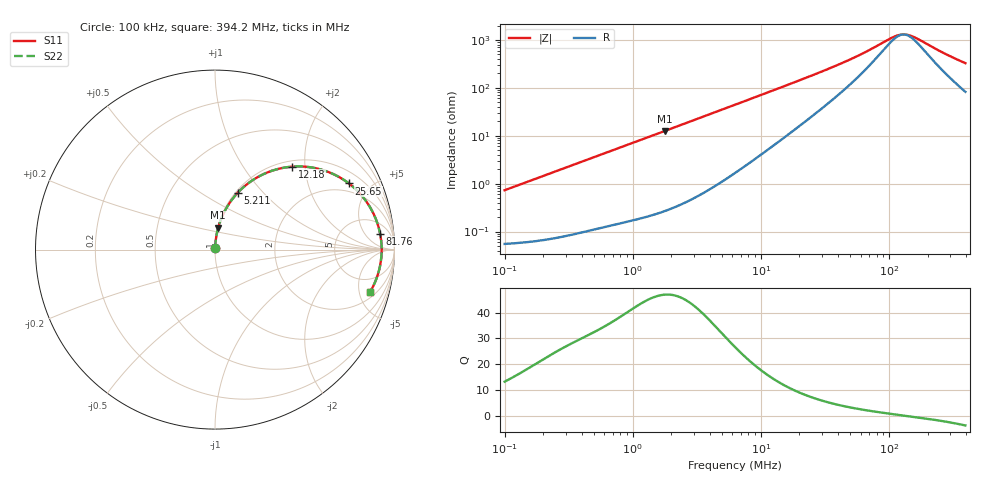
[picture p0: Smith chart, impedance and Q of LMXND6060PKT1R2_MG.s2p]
! LMXND6060PKT1R2_MG  S-PARAMETER MODEL  ( General Type )
! Model Generated by TAIYO YUDEN Corporation (https://www.yuden.co.jp/en/)
! Version 1.0
! TAIYO YUDEN Control No. 191025NI43SB-FBB
! Copyright(c) 2019 TAIYO YUDEN CO.,LTD. All Rights Reserved.
! Product Description (link to TY-COMPAS)
! https://ds.yuden.co.jp/TYCOMPAS/or/detail?pn=LMXND6060PKT1R2NMG&u=M
! Products Name : Inductors
! Characteristics :
!  Inductance : 1.2 uH , SRF(min) : 77 MHz , DC Resistance(max) : 0.0504 Ohm
!  Rated Current : Saturation :4000 mA , Temp Rise : 2750 mA (40 degC)
!  Case Size : 6.0 x 6.0 / 0.236 x 0.236 [mm/inch] , Thickness : 1.4 / 0.055 [mm/inch]
!  (Conditions: Temperature = 25 degC , DC Bias Current/Voltage = 0A / 0V)
! External Node Assignments :
!  1  o---GGG---o  2
! GND o---------o GND
! Frequency Range : 0.1MHz  -  394.189695MHz  [ 402 STEP ]
# MHz S RI R 50
! Freq[MHz].  S11 Real  S11 Imag  S21 Real  S21 Imag  S12 Real  S12 Imag  S22 Real  S22 Imag
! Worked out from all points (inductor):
!   401 points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, 100 kHz to 394.2 MHz, reference 50 ohm
!   read as one part in series: L = 1.15 uH near 104.2 kHz
!   highest Q = 47 at 1.776 MHz (marker M1), where L = 1.12 uH
!   self-resonance near 129.9 MHz
!   S11 on the Smith chart (normalised r, x): 100 kHz: 1.00, +0.01; 5.211 MHz: 1.02, +0.73; 12.18 MHz: 1.12, +1.72; 25.65 MHz: 1.54, +3.68; 81.76 MHz: 10, +12; 394.2 MHz: 2.65, -6.33
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0.1  0.000603 0.00724  0.9994 -0.00724  0.9994 -0.00724  0.000603 0.00724
0.400203  0.00177 0.0286  0.9982 -0.0286  0.9982 -0.0286  0.00177 0.0286
0.860763  0.00524 0.0606  0.9948 -0.0606  0.9948 -0.0606  0.00524 0.0606
1.601627  0.0149 0.1111  0.9851 -0.1111  0.9851 -0.1111  0.0149 0.1111
1.776264  0.018 0.1227  0.982 -0.1227  0.982 -0.1227  0.018 0.1227
3.237399  0.0542 0.2146  0.9458 -0.2146  0.9458 -0.2146  0.0542 0.2146
5.211338  0.1268 0.3169  0.8732 -0.3169  0.8732 -0.3169  0.1268 0.3169
6.278453  0.1731 0.36  0.8269 -0.36  0.8269 -0.36  0.1731 0.36
8.564294  0.2776 0.4239  0.7224 -0.4239  0.7224 -0.4239  0.2776 0.4239
12.17612  0.4314 0.4623  0.5686 -0.4623  0.5686 -0.4623  0.4314 0.4623
16.95654  0.5859 0.4475  0.4141 -0.4475  0.4141 -0.4475  0.5859 0.4475
25.12657  0.7395 0.3735  0.2605 -0.3735  0.2605 -0.3735  0.7395 0.3735
25.65208  0.7462 0.3685  0.2538 -0.3685  0.2538 -0.3685  0.7462 0.3685
43.0382  0.8642 0.2357  0.1358 -0.2357  0.1358 -0.2357  0.8642 0.2357
59.93525  0.9015 0.1561  0.0985 -0.1561  0.0985 -0.1561  0.9015 0.1561
81.75631  0.9198 0.0896  0.0802 -0.0896  0.0802 -0.0896  0.9198 0.0896
100.5574  0.926 0.0487  0.074 -0.0487  0.074 -0.0487  0.926 0.0487
123.682  0.9285 0.00923  0.0715 -0.00923  0.0715 -0.00923  0.9285 0.00923
145.9556  0.928 -0.022  0.072 0.022  0.072 0.022  0.928 -0.022
165.2556  0.9263 -0.0457  0.0737 0.0457  0.0737 0.0457  0.9263 -0.0457
277.2604  0.9027 -0.1527  0.0973 0.1527  0.0973 0.1527  0.9027 -0.1527
394.1897  0.8634 -0.2372  0.1366 0.2372  0.1366 0.2372  0.8634 -0.2372
